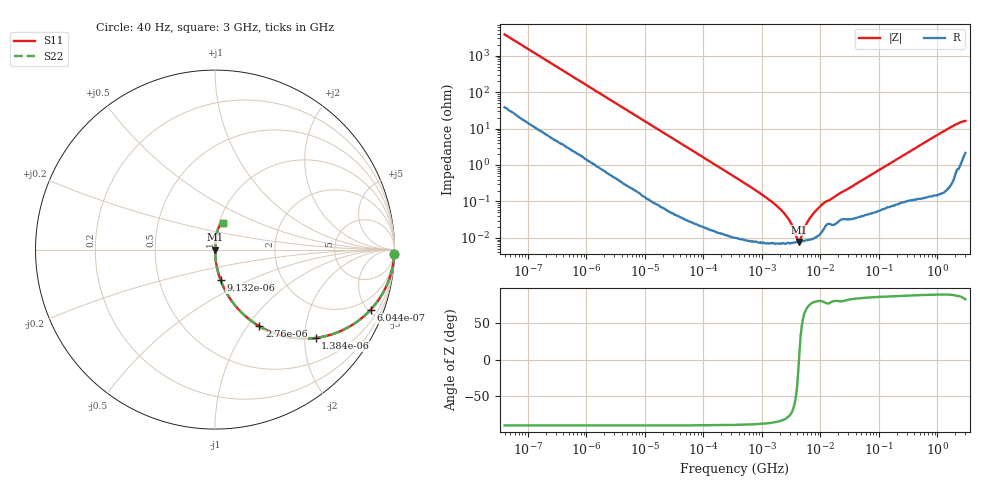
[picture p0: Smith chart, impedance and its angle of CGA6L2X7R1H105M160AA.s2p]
! S-parameter Generated by TDK Corporation
! Copyright(C) 2015 TDK Corporation.
! All Rights Reserved.
! TDK P/N: CGA6L2X7R1H105M160AA (Multilayer Ceramic Chip Capacitors)
! Property: C=1uF
! Size(LxWxT): 3.2x2.5x1.6mm, 0.126x0.098x0.063inches
! Model Type: s2p (Touchstone File Format Version 1.0)
! Frequency: DC=Yes Start=0.00004MHz Stop=3000MHz 396points Log-sweep
! Note: This model was converted from impedance.
! Model Generated on Jun. 23, 2015
! Hash(MD5):
! Port Assignments:
!  1 ---| |--- 2
! Applicable Conditions:
!  Temperature = 25 degC
!  DC Bias Voltage = 0 V
!  Small Signal Operation
! Terms and conditions regarding TDK Simulation Models
! (1)This simulation model is being provided solely for informational purposes. Please refer to the specifications of the products in terms of detailed characteristics of such products.
! (2)In no event shall TDK Corporation of any of its subsidiaries be liable for any loss or damage arising, directly or indirectly,
!  From any information contained in this simulation model, including, but not limited to loss or damages arising from any inaccuracies, omissions or errors in connection with such information.
! (3)Any and all copyrights on this simulation model are owned by TDK Corporation.
!  Duplication or redistribution of this simulation model without prior written permission from TDK Corporation is prohibited.
! (4)This simulation model is subject to any modification or change without any prior notice.
! (5)Neither TDK Corporation nor any of its subsidiaries shall make any warranty, express or implied,
!  Including but not limited to the correctness, implied warranties of merchantability and fitness for a particular purpose with respect to this simulation models.
! (6)The use of this simulation model shall be deemed to have consented to the terms and conditions hereof.
# MHz S MA R 50
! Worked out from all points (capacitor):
!   395 points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, 40 Hz to 3 GHz, reference 50 ohm
!   read as one part in series: C = 1.04 uF near 41.88 Hz
!   lowest |Z| = 7.77 mohm at 4.354 MHz (marker M1)
!   series resonance near 4.304 MHz, so ESL is about 1.3 nH
!   S11 on the Smith chart (normalised r, x): 40 Hz: 2, -76; 604.4 Hz: 1.05, -5.15; 1.384 kHz: 1.02, -2.26; 2.76 kHz: 1.01, -1.14; 9.132 kHz: 1.00, -0.35; 3 GHz: 1.04, +0.32
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4e-05  0.9994 -1.5  0.02618 87.9  0.02618 87.9  0.9994 -1.5
0.0001826612  0.992 -6.7  0.1171 82.8  0.1171 82.8  0.992 -6.7
0.0006043944  0.9294 -21.1  0.3606 68.3  0.3606 68.3  0.9294 -21.1
0.000834128  0.8785 -28.0  0.4697 61.5  0.4697 61.5  0.8785 -28.0
0.001383868  0.746 -41.2  0.6593 48.2  0.6593 48.2  0.746 -41.2
0.002759985  0.4932 -60.0  0.8656 29.6  0.8656 29.6  0.4932 -60.0
0.004794644  0.3121 -71.3  0.9474 18.2  0.9474 18.2  0.3121 -71.3
0.009132315  0.1712 -79.7  0.9838 9.9  0.9838 9.9  0.1712 -79.7
0.01739424  0.09141 -84.3  0.995 5.2  0.995 5.2  0.09141 -84.3
0.3464102  0.004675 -88.5  0.9999 0.3  0.9999 0.3  0.004675 -88.5
1.901634  0.0006963 -84.2  0.9999 0.0  0.9999 0.0  0.0006963 -84.2
2.877491  0.0003211 -76.9  0.9999 0.0  0.9999 0.0  0.0003211 -76.9
3.303516  0.0002142 -70.2  0.9999 0.0  0.9999 0.0  0.0002142 -70.2
3.971241  9.898e-05 -38.7  0.9999 0.0  0.9999 0.0  9.898e-05 -38.7
4.354128  7.773e-05 6.3  0.9999 -0.0  0.9999 -0.0  7.773e-05 6.3
4.5592  9.27e-05 30.6  0.9999 -0.0  0.9999 -0.0  9.27e-05 30.6
5.738865  0.0002405 68.9  0.9999 -0.0  0.9999 -0.0  0.0002405 68.9
7.22376  0.000426 77.3  0.9999 -0.0  0.9999 -0.0  0.000426 77.3
11.98465  0.000959 77.8  0.9998 -0.1  0.9998 -0.1  0.000959 77.8
150.6385  0.01081 85.7  0.9992 -0.6  0.9992 -0.6  0.01081 85.7
1575.059  0.1019 82.8  0.9924 -5.8  0.9924 -5.8  0.1019 82.8
3000  0.1564 73.4  0.9671 -8.9  0.9671 -8.9  0.1564 73.4
